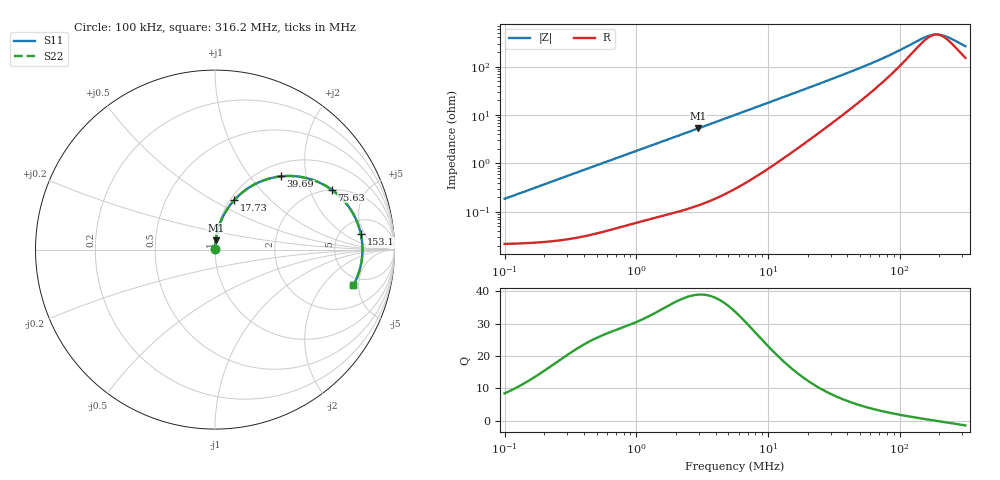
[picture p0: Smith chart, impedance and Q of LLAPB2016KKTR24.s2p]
! LLAPB2016KKTR24  S-PARAMETER MODEL  ( General Type )
! Model Generated by TAIYO YUDEN Corporation (http://www.ty-top.com)
! Version 1.0
! TAIYO YUDEN Control No. 151002NG33SB-FKC
! Copyright(c) 2015 TAIYO YUDEN CO.,LTD. All Rights Reserved.
! Product Description (link to TY-COMPAS)
! https://ds.yuden.co.jp/TYCOMPAS/or/detail?pn=LLAPB2016KKTR24M&u=M
! Products Name : Inductors
! Characteristics :
!  Inductance : 0.24 uH , SRF(min) : -Hz , DC Resistance(max) : 0.026 Ohm
!  Rated Current : Saturation :5800 mA , Temp Rise : 4000 mA (40 degC)
!  Case Size : 2.0 x 1.6 / 0.079 x 0.063 [mm/inch] , Thickness : 1 / 0.039 [mm/inch]
!  (Conditions: Temperature = 25 degC , DC Bias Current/Voltage = 0A / 0V)
! External Node Assignments :
!  1  o---GGG---o  2
! GND o---------o GND
! Frequency Range : 0.1MHz  -  316.199832MHz  [ 402 STEP ]
# MHz S RI R 50
! Freq[MHz].  S11 Real  S11 Imag  S21 Real  S21 Imag  S12 Real  S12 Imag  S22 Real  S22 Imag
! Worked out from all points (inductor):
!   401 points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, 100 kHz to 316.2 MHz, reference 50 ohm
!   read as one part in series: L = 293 nH near 104.1 kHz
!   highest Q = 39 at 2.951 MHz (marker M1), where L = 284 nH
!   self-resonance near 190.7 MHz
!   S11 on the Smith chart (normalised r, x): 100 kHz: 1.00, +0.00; 17.73 MHz: 1.05, +0.63; 39.69 MHz: 1.23, +1.44; 75.63 MHz: 1.99, +2.85; 153.1 MHz: 7.78, +4.07; 316.2 MHz: 4.02, -4.33
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0.1  0.000221 0.00184  0.9998 -0.00184  0.9998 -0.00184  0.000221 0.00184
0.385695  0.000355 0.00707  0.9996 -0.00707  0.9996 -0.00707  0.000355 0.00707
1.487603  0.0015 0.0267  0.9985 -0.0267  0.9985 -0.0267  0.0015 0.0267
2.9511  0.00411 0.0524  0.9959 -0.0524  0.9959 -0.0524  0.00411 0.0524
5.623165  0.0128 0.0987  0.9872 -0.0987  0.9872 -0.0987  0.0128 0.0987
10.93271  0.0447 0.1846  0.9553 -0.1846  0.9553 -0.1846  0.0447 0.1846
17.73068  0.1079 0.2765  0.8921 -0.2765  0.8921 -0.2765  0.1079 0.2765
21.68824  0.1524 0.3185  0.8476 -0.3185  0.8476 -0.3185  0.1524 0.3185
28.75564  0.2379 0.3721  0.7621 -0.3721  0.7621 -0.3721  0.2379 0.3721
39.69369  0.3675 0.4081  0.6325 -0.4081  0.6325 -0.4081  0.3675 0.4081
46.63594  0.4406 0.4094  0.5594 -0.4094  0.5594 -0.4094  0.4406 0.4094
54.79236  0.5146 0.3973  0.4854 -0.3973  0.4854 -0.3973  0.5146 0.3973
75.63424  0.65 0.334  0.35 -0.334  0.35 -0.334  0.65 0.334
83.65039  0.6857 0.3053  0.3143 -0.3053  0.3143 -0.3053  0.6857 0.3053
113.1661  0.7682 0.2028  0.2318 -0.2028  0.2318 -0.2028  0.7682 0.2028
153.0964  0.8125 0.087  0.1875 -0.087  0.1875 -0.087  0.8125 0.087
165.9452  0.8181 0.0552  0.1819 -0.0552  0.1819 -0.0552  0.8181 0.0552
179.8723  0.8212 0.0232  0.1788 -0.0232  0.1788 -0.0232  0.8212 0.0232
191.0795  0.8218 -0.000839  0.1782 0.000839  0.1782 0.000839  0.8218 -0.000839
207.116  0.8205 -0.0329  0.1795 0.0329  0.1795 0.0329  0.8205 -0.0329
233.7293  0.8138 -0.0807  0.1862 0.0807  0.1862 0.0807  0.8138 -0.0807
316.1998  0.7715 -0.197  0.2285 0.197  0.2285 0.197  0.7715 -0.197
